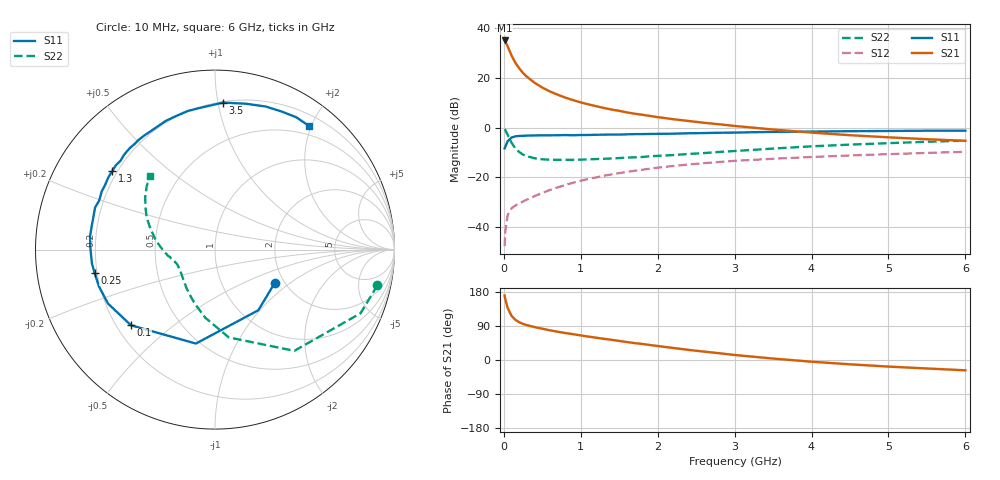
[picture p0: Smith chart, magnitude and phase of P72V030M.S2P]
! SIEMENS Small Signal Semiconductors
! BFP196
! Si NPN RF Bipolar Junction Transistor in SOT143
! VCE = 2 V  IC = 30 mA
! Common Emitter S-Parameters:  May  1996
# GHz  S  MA  R  50
!  f  S11  S21  S12  S22
! GHz  MAG  ANG  MAG  ANG  MAG  ANG  MAG  ANG
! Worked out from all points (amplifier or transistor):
!   36 points, 10 MHz to 6 GHz, reference 50 ohm
!   highest |S21| = 34.9 dB at 10 MHz (marker M1)
!   |S21| within 3 dB of that: start of sweep to 58.4 MHz
!   unconditionally stable (mu >= 1): 536 MHz to 4.295 GHz
!   at 250 MHz: K = 0.74, MSG = 25.7 dB, |S12| = -29.6 dB
!   at 1.4 GHz: K = 1.10, MAG = 11.1 dB, |S12| = -18.8 dB
!   at 6 GHz: K = 0.98, MSG = 2.2 dB, |S12| = -9.7 dB
!   lowest NFmin = 1.40 dB at 500 MHz
!   S11 on the Smith chart (normalised r, x): 10 MHz: 1.78, -0.78; 100 MHz: 0.26, -0.36; 250 MHz: 0.19, -0.09; 1.3 GHz: 0.18, +0.33; 3.5 GHz: 0.21, +1.03; 6 GHz: 0.36, +1.96
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0.01  0.3811 -29.4  55.64 170.2  0.0042 81.6  0.9265 -12.4
0.02  0.4152 -54.4  52.55 159.6  0.0086 74.5  0.8853 -23.6
0.05  0.5343 -101.5  42.27 137.2  0.0177 55.4  0.7167 -51.9
0.1  0.6302 -138.0  27.8 116.6  0.0241 46.0  0.4951 -81.1
0.15  0.6679 -153.3  19.89 106.1  0.0274 44.1  0.383 -98.2
0.2  0.6783 -162.4  15.4 99.6  0.0302 44.8  0.3225 -110.3
0.25  0.6834 -169.2  12.38 95.2  0.0331 46.3  0.286 -119.8
0.3  0.69 -173.5  10.41 91.9  0.036 48.7  0.2668 -126.5
0.4  0.6948 179.0  7.896 86.8  0.0423 52.4  0.2426 -136.8
0.5  0.7 174.0  6.329 82.5  0.0489 55.1  0.2315 -143.7
0.6  0.6994 169.0  5.28 78.3  0.0563 56.5  0.227 -148.6
0.7  0.7018 164.6  4.552 74.5  0.0633 57.5  0.2254 -152.4
0.9  0.7008 157.0  3.542 68.1  0.0784 57.5  0.225 -157.8
1.1  0.7105 149.5  2.917 61.7  0.0934 56.9  0.2309 -161.5
1.3  0.7207 142.7  2.471 55.9  0.1082 55.1  0.2367 -164.8
1.7  0.7383 130.1  1.896 44.6  0.1362 51.0  0.2534 -170.5
2.2  0.7537 116.6  1.471 31.8  0.1696 44.4  0.2812 -177.2
3  0.7928 96.8  1.077 13.2  0.2149 33.4  0.3388 169.8
3.5  0.8202 86.9  0.913 3.8  0.2371 26.9  0.3789 161.9
4.5  0.8457 70.5  0.703 -11.4  0.2761 15.2  0.4552 148.4
5.5  0.8654 58.4  0.584 -22.4  0.3106 4.4  0.5193 137.1
6  0.8654 52.8  0.543 -27.2  0.3264 -1.4  0.5483 131.5
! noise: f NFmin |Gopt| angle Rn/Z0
0.5  1.4  0.4  -173  0.08
0.9  1.6  0.5  -166  0.08
1.5  2.4  0.61  -150  0.14
2  2.9  0.71  -129  0.2
